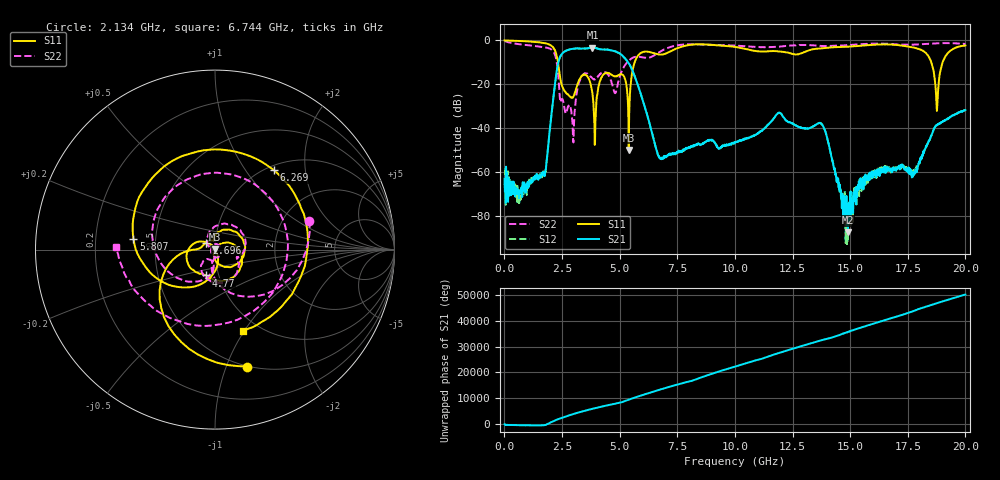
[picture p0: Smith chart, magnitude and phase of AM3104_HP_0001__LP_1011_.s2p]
!Created with skrf (http://scikit-rf.org).
# Hz S RI R 50.0
!freq ReS11 ImS11 ReS21 ImS21 ReS12 ImS12 ReS22 ImS22
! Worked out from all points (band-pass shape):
!   1601 points, 10 MHz to 20 GHz, reference 50 ohm
!   highest |S21| = -3.22 dB at 3.821 GHz (marker M1); lowest = -87.6 dB at 14.9 GHz (marker M2)
!   |S21| within 3 dB of the highest: 2.489 GHz to 5.045 GHz (2.556 GHz wide, 67.9 % of centre)
!   lowest |S11| = -49.9 dB at 5.395 GHz (marker M3), VSWR 1.01, Z = 50 + j0.315 ohm
!   |S11| at or under -10 dB: 2.324 GHz to 5.651 GHz (3.326 GHz wide, 83.4 % of centre); 18.52 GHz to 19.01 GHz (487.2 MHz wide, 2.6 % of centre)
!   |S22| runs from -46.5 to -0.2 dB; largest |S21 - S12| = 0.0048
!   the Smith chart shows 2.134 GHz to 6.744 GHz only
!   S11 on the Smith chart (normalised r, x): 2.134 GHz: 0.49, -1.19; 2.696 GHz: 0.91, +0.07; 4.77 GHz: 0.87, -0.26; 5.807 GHz: 0.37, +0.06; 6.269 GHz: 1.08, +1.37; 6.744 GHz: 0.84, -0.98
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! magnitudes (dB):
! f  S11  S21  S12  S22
! 10 MHz  0.0  -63.1  -66.1  -0.2
! 1.697 GHz  -1.1  -60.8  -60.4  -3.1
! 2.134 GHz  -3.4  -25.3  -25.3  -5.2
! 2.696 GHz  -24.1  -4.6  -4.5  -32.6
! 2.996 GHz  -25.6  -3.7  -3.7  -46.5
! 3.346 GHz  -16.2  -3.7  -3.7  -16.5
! 3.821 GHz  -24.2  -3.2  -3.2  -17.3
! 4.77 GHz  -16.4  -4.9  -4.9  -23.7
! 5.395 GHz  -49.9  -10.4  -10.4  -9.2
! 5.807 GHz  -6.8  -20.9  -20.9  -7.4
! 6.269 GHz  -5.2  -36.8  -36.8  -7.9
! 6.682 GHz  -6.3  -52.6  -52.7  -5.6
! 6.744 GHz  -6.4  -53.8  -53.9  -5.1
! 10.01 GHz  -2.9  -46.6  -46.7  -2.3
! 13.34 GHz  -4.1  -39.5  -39.5  -2.2
! 13.87 GHz  -3.5  -40.0  -40.0  -2.5
! 14.9 GHz  -2.8  -87.6  -75.5  -2.1
! 16.68 GHz  -1.8  -58.3  -58.7  -1.5
! 18.28 GHz  -5.6  -49.2  -49.1  -1.6
! 18.76 GHz  -32.2  -38.7  -38.6  -1.3
! 19.15 GHz  -7.0  -36.1  -36.0  -1.2
! 20 GHz  -2.3  -31.8  -31.7  -1.6
